FUNCTION FC 10 : BOOL
TITLE =
VERSION : 0.1


VAR_INPUT
  Melder1 : BOOL ;
  Melder2 : BOOL ;
  Melder3 : BOOL ;
END_VAR
BEGIN
NETWORK
TITLE =
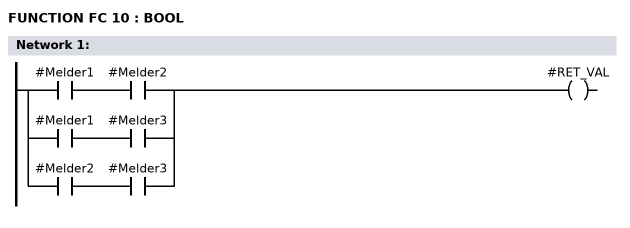
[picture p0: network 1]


      U     #Melder1;
      U     #Melder2;
      O     ;
      U     #Melder1;
      U     #Melder3;
      O     ;
      U     #Melder2;
      U     #Melder3;
      =     #RET_VAL;

END_FUNCTION

ORGANIZATION_BLOCK OB 1
TITLE = "Main Program Sweep (Cycle)"
VERSION : 0.1


VAR_TEMP
  OB1_EV_CLASS : BYTE ;	//Bits 0-3 = 1 (Coming event), Bits 4-7 = 1 (Event class 1)
  OB1_SCAN_1 : BYTE ;	//1 (Cold restart scan 1 of OB 1), 3 (Scan 2-n of OB 1)
  OB1_PRIORITY : BYTE ;	//1 (Priority of 1 is lowest)
  OB1_OB_NUMBR : BYTE ;	//1 (Organization block 1, OB1)
  OB1_RESERVED_1 : BYTE ;	//Reserved for system
  OB1_RESERVED_2 : BYTE ;	//Reserved for system
  OB1_PREV_CYCLE : INT ;	//Cycle time of previous OB1 scan (milliseconds)
  OB1_MIN_CYCLE : INT ;	//Minimum cycle time of OB1 (milliseconds)
  OB1_MAX_CYCLE : INT ;	//Maximum cycle time of OB1 (milliseconds)
  OB1_DATE_TIME : DATE_AND_TIME ;	//Date and time OB1 started
END_VAR
BEGIN
NETWORK
TITLE =

      CALL FC    10 (
           Melder1                  := E      0.1,
           Melder2                  := E      0.2,
           Melder3                  := E      0.3,
           RET_VAL                  := A      4.0);



END_ORGANIZATION_BLOCK

